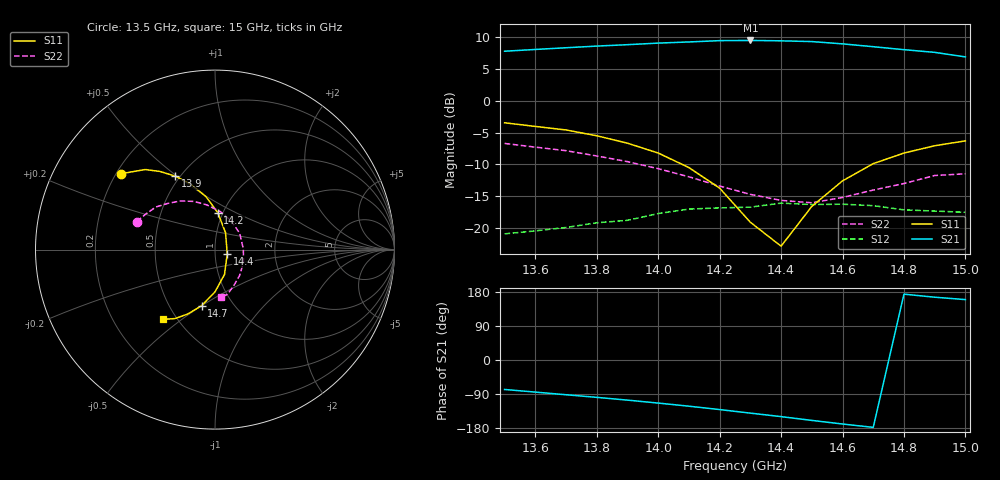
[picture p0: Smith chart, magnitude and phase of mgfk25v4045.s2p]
! MGFK25V4045  (Ta=25deg. C, VDS=8V, lDS=150mA)"
! Date=9 June 1999
# GHZ S MA R 50
!  Freq.  S11  S21  S12  S22
!  GHz  (mag)  (ang)  (mag)  (ang)  (mag)  (ang)  (mag)  (ang)
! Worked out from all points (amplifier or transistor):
!   16 points, 13.5 GHz to 15 GHz, reference 50 ohm
!   highest |S21| = 9.5 dB at 14.3 GHz (marker M1)
!   |S21| within 3 dB of that: start of sweep to end of sweep
!   unconditionally stable (mu >= 1): start of sweep to end of sweep
!   at 13.7 GHz: K = 1.35, MAG = 10.6 dB, |S12| = -19.9 dB
!   at 14.3 GHz: K = 1.31, MAG = 9.8 dB, |S12| = -16.7 dB
!   at 15 GHz: K = 1.43, MAG = 8.3 dB, |S12| = -17.5 dB
!   S11 on the Smith chart (normalised r, x): 13.5 GHz: 0.22, +0.34; 13.9 GHz: 0.47, +0.49; 14.2 GHz: 0.95, +0.41; 14.4 GHz: 1.15, -0.05; 14.7 GHz: 0.72, -0.50; 15 GHz: 0.42, -0.43
13.5  0.673 141.1  2.46 -77.8  0.09 -125.1  0.463 160.3
13.6  0.63 136.4  2.54 -84.7  0.095 -131.2  0.433 152.6
13.7  0.591 131.0  2.62 -91.7  0.101 -135.1  0.406 144.2
13.8  0.532 125.1  2.7 -98.6  0.11 -141.9  0.369 135.9
13.9  0.465 118.4  2.77 -105.9  0.115 -153.0  0.333 125.5
14  0.389 110.3  2.85 -113.7  0.13 -159.4  0.293 113.6
14.1  0.299 99.6  2.91 -121.9  0.141 -167.1  0.253 100.3
14.2  0.206 85.6  2.98 -130.8  0.144 -176.4  0.214 82.1
14.3  0.111 58.1  2.99 -140.2  0.146 174.9  0.184 60.8
14.4  0.072 -18.6  2.97 -149.4  0.157 163.4  0.165 33.8
14.5  0.148 -69.0  2.93 -159.4  0.153 155.7  0.158 1.6
14.6  0.235 -89.9  2.81 -168.9  0.154 146.5  0.174 -24.3
14.7  0.321 -103.4  2.67 -177.8  0.15 136.6  0.199 -46.4
14.8  0.389 -112.8  2.53 173.8  0.139 129.3  0.224 -61.4
14.9  0.444 -120.1  2.41 165.7  0.136 121.8  0.259 -74.4
15  0.485 -126.6  2.22 159.4  0.133 118.0  0.267 -82.5
